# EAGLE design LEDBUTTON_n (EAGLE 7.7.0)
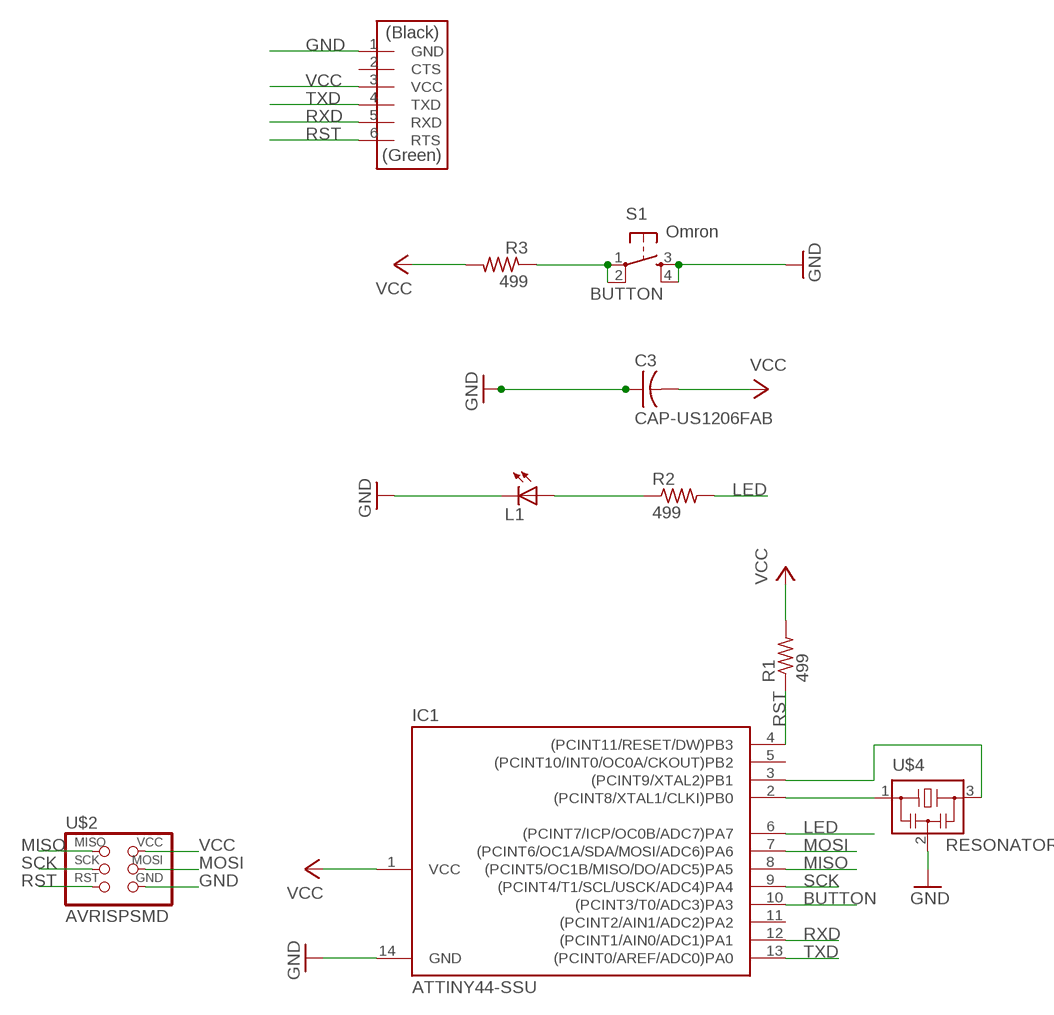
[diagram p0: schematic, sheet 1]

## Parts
C3  CAP-US1206FAB  [C1206FAB]
IC1  ATTINY44-SSU  [SOIC14]
L1  LEDFAB1206  [LED1206FAB]
R1  499  RES-US1206FAB  [R1206FAB]
R2  499  RES-US1206FAB  [R1206FAB]
R3  499  RES-US1206FAB  [R1206FAB]
S1  Omron  6MM_SWITCH6MM_SWITCH  [6MM_SWITCH]
U$1  FTDI-SMD-HEADER  [1X06SMD]
U$2  AVRISPSMD  [2X03SMD]
U$4  RESONATOR  [EFOBM]

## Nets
BUTTON: IC1.10((PCINT3/T0/ADC3)PA3) R3.1 S1.1(P) S1.2(P1)
GND: C3.1 IC1.14(GND) L1.2(C) S1.3(S) S1.4(S1) U$1.1(GND) U$2.6(GND) U$4.2
LED: IC1.6((PCINT7/ICP/OC0B/ADC7)PA7) R2.2
MISO: IC1.8((PCINT5/OC1B/MISO/DO/ADC5)PA5) U$2.1(MISO)
MOSI: IC1.7((PCINT6/OC1A/SDA/MOSI/ADC6)PA6) U$2.4(MOSI)
N$1: IC1.2((PCINT8/XTAL1/CLKI)PB0) U$4.1
N$2: IC1.3((PCINT9/XTAL2)PB1) U$4.3
N$3: L1.1(A) R2.1
RST: IC1.4((PCINT11/RESET/DW)PB3) R1.1 U$1.6(RTS) U$2.5(RST)
RXD: IC1.12((PCINT1/AIN0/ADC1)PA1) U$1.5(RXD)
SCK: IC1.9((PCINT4/T1/SCL/USCK/ADC4)PA4) U$2.3(SCK)
TXD: IC1.13((PCINT0/AREF/ADC0)PA0) U$1.4(TXD)
VCC: C3.2 IC1.1(VCC) R1.2 R3.2 U$1.3(VCC) U$2.2(VCC)
Unconnected: IC1.5((PCINT10/INT0/OC0A/CKOUT)PB2) IC1.11((PCINT2/AIN1/ADC2)PA2) U$1.2(CTS)

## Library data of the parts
C3 = fab:CAP-US
IC1 = fab:ATTINY44
L1 = fab:LED: LED
R1-R3 = fab:RES-US: Resistor (US Symbol)
S1 = fab:6MM_SWITCH: OMRON SWITCH
U$1 = fab:FTDI-SMD-HEADER
U$2 = fab:AVRISP
U$4 = fab:RESONATOR

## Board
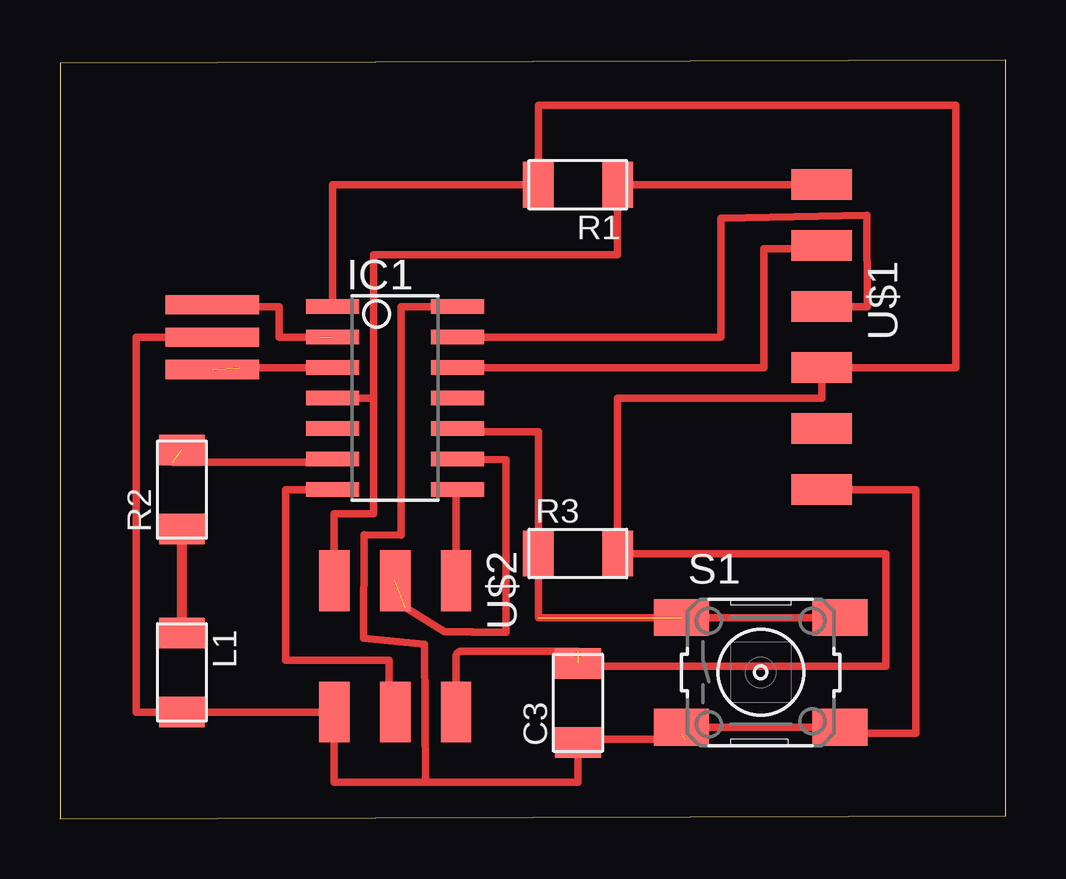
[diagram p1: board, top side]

Size 39.42 x 31.61 mm. Coordinates in mm from the lower left corner, seen from the top.
Outline: 0,0 39.42,0.13 39.42,31.61 0,31.49 0,0
Copper layers (1*16): Top 0.035mm / dielectric 1.5mm / Bottom 0.035mm
Design rules "default *": minimum track width 10mil, minimum drill 24mil, track to track 16mil, track to pad 16mil, pad to pad 16mil, via to via 16mil, smd to smd 8mil, copper to edge 40mil, drill to drill 8mil, minimum pad ring 10mil, minimum via ring 8mil, stop-mask expansion 4mil, vias tented up to drill 0mil, thermal gap 10mil

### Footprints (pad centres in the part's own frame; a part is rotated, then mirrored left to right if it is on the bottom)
C1206FAB = smd 1.27 x 1.905: 1 -1.651,0; 2 1.651,0
SOIC14 = smd 0.61 x 2.21: 1 -3.81,-2.603; 2 -2.54,-2.603; 3 -1.27,-2.603; 4 0,-2.603; 5 1.27,-2.603; 6 2.54,-2.603; 7 3.81,-2.603; 8 3.81,2.603; 9 2.54,2.603; 10 1.27,2.603; 11 0,2.603; 12 -1.27,2.603; 13 -2.54,2.603; 14 -3.81,2.603
LED1206FAB = smd 1.27 x 1.905: 1 -1.651,0; 2 1.651,0
R1206FAB = smd 1.27 x 1.905: 1 -1.651,0; 2 1.651,0
6MM_SWITCH = smd 2.286 x 1.524: 1 -3.302,2.286; 2 3.302,2.286; 3 -3.302,-2.286; 4 3.302,-2.286
1X06SMD = smd 2.54 x 1.27: 1 0,6.35; 2 0,3.81; 3 0,1.27; 4 0,-1.27; 5 0,-3.81; 6 0,-6.35
2X03SMD = smd 2.54 x 1.27: 1 -2.54,2.54; 2 2.92,2.54; 3 -2.54,0; 4 2.92,0; 5 -2.54,-2.54; 6 2.92,-2.54
EFOBM = smd 0.8 x 3.9: 1 -1.35,0; 2 0,0; 3 1.35,0

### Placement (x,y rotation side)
C3  21.59,4.83 90 top
IC1  13.97,17.53 270 top
L1  5.08,6.1 270 top
R1  21.59,26.42 180 top
R2  5.08,13.72 90 top
R3  21.59,11.05 0 top
S1  29.21,6.1 0 top
U$1  31.75,20.07 180 top
U$2  13.97,7.37 270 top
U$4  6.35,20.07 270 top

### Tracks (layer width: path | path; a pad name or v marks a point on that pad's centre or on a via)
BUTTON  (1 unrouted)
  Top 0.305: IC1.10 16.57,16.13 19.94,16.13 R3.1 19.94,8.38 S1.2
GND  (1 unrouted)
  Top 0.254: 15.85,21.39 16.51,21.39 IC1.14
  Top 0.305: 15.85,21.39 15.85,21.34 14.22,21.34 14.22,11.81 12.67,11.84 12.65,7.52 15.19,7.26 15.24,1.52 | U$4.2 3.18,20.07 3.18,4.45 L1.2 | 25.91,3.56 S1.3 S1.4 32.51,3.56 35.69,3.56 35.69,13.72 U$1.1 | 5.46,4.45 U$2.6 11.43,1.52 15.24,1.52 | 21.59,3.56 21.59,3.3 26.04,3.3 | 15.24,1.52 21.59,1.52 C3.1
  Top 0.406: L1.2 5.08,4.83 5.46,4.45 | 16.51,21.34 IC1.14 | C3.1 21.59,3.56
LED  (1 unrouted)
  Top 0.305: IC1.6 11.37,14.86 4.7,14.86
MISO
  Top 0.254: 16.66,13.56 IC1.8 | 16.66,9.93 U$2.1
  Top 0.305: IC1.8 arc90 16.51,13.65 U$2.1
MOSI
  Top 0.305: IC1.7 9.4,13.72 9.4,6.6 13.72,6.6 13.72,4.45 U$2.4
N$1  (1 unrouted)
  Top 0.305: U$4.1 6.35,21.34 9.14,21.34 9.14,20.07 10.79,20.07
N$2  (1 unrouted)
  Top 0.305: IC1.3 7.49,18.8
N$3
  Top 0.406: R2.1 L1.1
RST
  Top 0.305: U$1.6 R1.1 23.24,23.49 13.08,23.49 13.08,17.53 | U$2.5 11.43,12.7 13.08,12.7 13.08,17.53 | IC1.4 13.08,17.53
RXD
  Top 0.305: U$1.5 31.75,23.75 29.34,23.75 29.34,18.8 IC1.12
SCK  (1 unrouted)
  Top 0.305: IC1.9 18.59,14.96 18.59,7.77 17.17,7.77 17.17,7.8 16.03,7.8 14.38,8.81
TXD
  Top 0.305: U$1.4 33.66,21.34 33.63,25.15 27.56,25.02 27.56,20.07 IC1.13
VCC  (1 unrouted)
  Top 0.254: 21.29,6.3 C3.2 | 16.66,4.65 U$2.2
  Top 0.305: 21.29,6.3 arc90 21.36,6.22 | 16.66,4.65 arc-90 16.51,4.8 16.51,6.73 arc-90 16.76,6.99 21.59,6.99 | C3.2 21.59,6.35 34.42,6.35 34.42,11.05 R3.2 23.24,17.53 31.75,17.53 U$1.3 37.34,18.8 37.34,29.72 19.94,29.72 R1.2 11.37,26.42 IC1.1
  Top 0.406: 11.05,21.34 IC1.1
